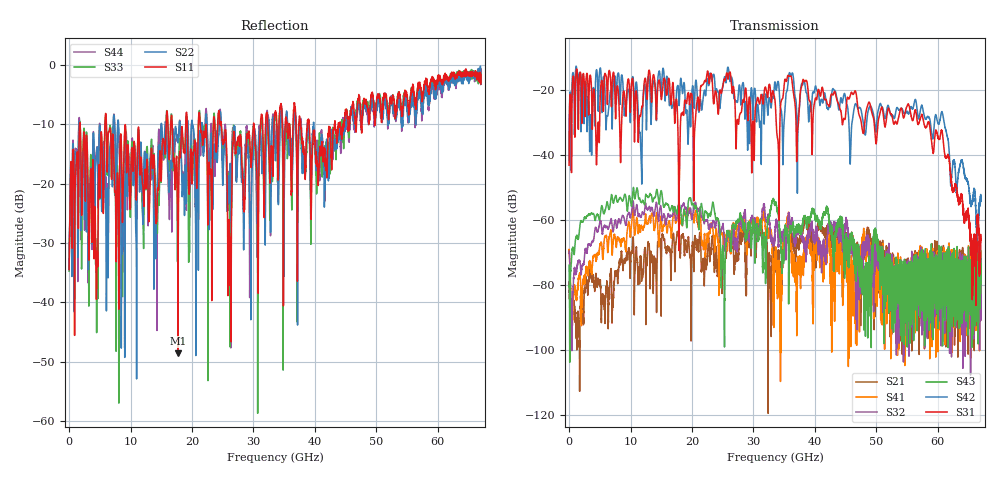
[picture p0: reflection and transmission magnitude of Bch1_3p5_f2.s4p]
!Agilent Technologies,N5247A,US51170199,A.09.90.13
!Agilent N5247A: A.09.90.13
!Date: Thursday, October 18, 2018 09:59:48
!Correction: S11(Full 4 Port(1,2,3,4))
!S12(Full 4 Port(1,2,3,4))
!S13(Full 4 Port(1,2,3,4))
!S14(Full 4 Port(1,2,3,4))
!S21(Full 4 Port(1,2,3,4))
!S22(Full 4 Port(1,2,3,4))
!S23(Full 4 Port(1,2,3,4))
!S24(Full 4 Port(1,2,3,4))
!S31(Full 4 Port(1,2,3,4))
!S32(Full 4 Port(1,2,3,4))
!S33(Full 4 Port(1,2,3,4))
!S34(Full 4 Port(1,2,3,4))
!S41(Full 4 Port(1,2,3,4))
!S42(Full 4 Port(1,2,3,4))
!S43(Full 4 Port(1,2,3,4))
!S44(Full 4 Port(1,2,3,4))
!S4P File: Measurements: <S11,S12,S13,S14>,
!<S21,S22,S23,S24>,
!<S31,S32,S33,S34>,
!<S41,S42,S43,S44>:
# Hz S  dB  R 50
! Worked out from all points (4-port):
!   6701 points, 10 MHz to 67 GHz, reference 50 ohm
!   strongest paths, dB at 10 MHz, 16.76 GHz, 33.51 GHz, 50.25 GHz, 67 GHz:
!     S31: -43.1, -20.3, -23.3, -30.4, -67.1
!     S42: -41.7, -25.5, -17.5, -26.6, -53.7
!     S43: -73.9, -55.7, -55.3, -68.6, -69.6
!     S32: -69.6, -58.7, -63.5, -70.6, -75.5
!     S41: -70.1, -62.7, -73.3, -73.5, -72.6
!     S21: -80.2, -68.1, -69.7, -73.3, -80.1
!   lowest |S11| = -48.5 dB at 17.73 GHz (marker M1), VSWR 1.01, Z = 49.6 - j0.11 ohm
!   |S11| at or under -10 dB: 6.073 GHz to 15.79 GHz (9.716 GHz wide, 88.9 % of centre); 24.77 GHz to 30.01 GHz (5.243 GHz wide, 19.1 % of centre); 39.05 GHz to 43.21 GHz (4.16 GHz wide, 10.1 % of centre)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
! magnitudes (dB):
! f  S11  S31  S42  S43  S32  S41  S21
! 10 MHz  -34.5  -43.1  -41.7  -73.9  -69.6  -70.1  -80.2
! 13.04 GHz  -25.6  -13.9  -16.9  -52.6  -56.0  -59.4  -67.4
! 17.73 GHz  -48.5  -33.7  -18.6  -55.9  -56.5  -56.9  -64.6
! 22.77 GHz  -16.7  -17.6  -18.1  -58.3  -62.7  -64.2  -66.5
! 33.99 GHz  -19.4  -35.9  -17.4  -57.8  -65.0  -77.0  -70.5
! 55.15 GHz  -7.1  -24.4  -27.1  -91.0  -73.7  -77.4  -93.6
! 67 GHz  -3.3  -67.1  -53.7  -69.6  -75.5  -72.6  -80.1
